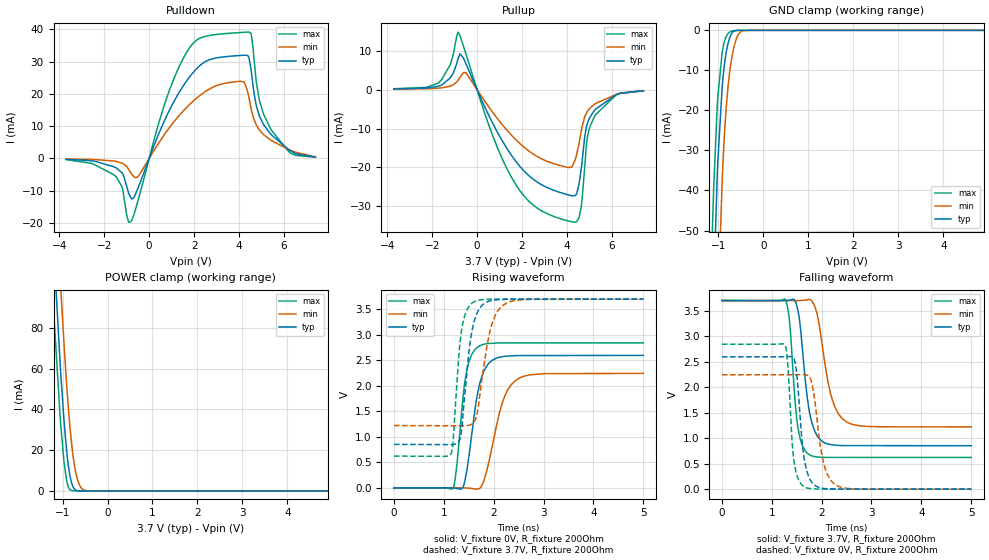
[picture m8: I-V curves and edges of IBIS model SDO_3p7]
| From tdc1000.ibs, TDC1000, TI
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|   Model
[Model]   SDO_3p7
Model_type   I/O
Polarity   Non-Inverting
Enable   Active-Low
Vinl = 1.11
Vinh = 2.59
Vmeas = 1.85
Vref = 0
Cref = 1pF
Rref = 100000
|   typ   min   max
C_comp   0.670pF   0.613pF   0.704pF
[Voltage Range]   3.7   3.699   3.701
[Temperature Range]   27   125   -40
[Pullup Reference]   3.7   3.699   3.701
[Pulldown Reference]   0   0   0
[Power Clamp Reference]   3.7   3.699   3.701
[GND Clamp Reference]   0   0   0
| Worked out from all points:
|   slope of the pulldown table from 0 to 0.555 V, typ, clamps not added: 57.1 ohm
|   slope of the pullup table from 0 to 0.555 V, typ, clamps not added: 79.3 ohm
|   GND clamp passes 1 mA (typ) near -0.71 V on its own axis
|   POWER clamp passes 1 mA (typ) near -0.74 V on its own axis
|   falling waveform, V_fixture 3.7V, R_fixture 200Ohm: 20-80 % time 197ps typ, 272ps min, 146ps max; typ from 3.7 V to 0.852 V
|   rising waveform, V_fixture 0V, R_fixture 200Ohm: 20-80 % time 241ps typ, 331ps min, 182ps max; typ from 0 V to 2.6 V
|   rising waveform, V_fixture 3.7V, R_fixture 200Ohm: 20-80 % time 193ps typ, 254ps min, 148ps max; typ from 0.852 V to 3.7 V
|   falling waveform, V_fixture 0V, R_fixture 200Ohm: 20-80 % time 148ps typ, 202ps min, 110ps max; typ from 2.6 V to 0 V
[Pulldown]
|   Voltage   I(typ)   I(min)   I(max)
-3.7V     -264.4uA   -158.9uA   -366.5uA
-1.491V   -2.825mA   -880.5uA   -5.512mA
-802.9mV  -12.37mA   -4.609mA   -19.5mA
640.1mV   11.08mA    7.012mA    15.79mA
1.728V    24.59mA    16.25mA    33.56mA
3.282V    31.44mA    23.14mA    38.61mA
4.381V    31.9mA     20.72mA    39.15mA
4.547V    26.85mA    15.15mA    38.38mA
4.769V    16.29mA    10.36mA    23.54mA
5.413V    7.511mA    5.656mA    9.091mA
6.334V    2.177mA    2.404mA    1.482mA
7.4V      424.2uA    504.5uA    390.1uA
[GND Clamp]
|   Voltage   I(typ)   I(min)   I(max)
-3.7V     -1.666A    -1.714A    -1.629A
-1.136V   -79.36mA   -127.2mA   -51.21mA
-1.125V   -74.22mA   -121.7mA   -46.88mA
-1.103V   -64.39mA   -110.8mA   -39mA
-1.014V   -33.13mA   -70.93mA   -16.92mA
-913.9mV  -13.9mA    -37.2mA    -5.349mA
-891.7mV  -11.24mA   -31.74mA   -4.004mA
-825.1mV  -5.503mA   -19.3mA    -1.54mA
-725.2mV  -1.216mA   -8.495mA   -302.2uA
-603.1mV  -61.85uA   -2.248mA   -21.83uA
-447.7mV  -847.8nA   -90.96uA   -178.6nA
7.4V      0A         0A         0A
[Pullup]
|   Voltage   I(typ)   I(min)   I(max)
-3.7V     166.1uA    103uA      227.5uA
-1.724V   857.1uA    384uA      1.69mA
-1.191V   3.033mA    905.6uA    6.459mA
-847.3mV  7.891mA    2.377mA    14.78mA
-492.1mV  6.622mA    4.285mA    9.107mA
640.1mV   -7.998mA   -5.394mA   -10.97mA
1.728V    -18.45mA   -12.87mA   -24.43mA
4.37V     -27.23mA   -17.96mA   -34.06mA
4.625V    -20.84mA   -11.02mA   -30.52mA
4.902V    -8.802mA   -5.659mA   -12.56mA
5.191V    -5.588mA   -3.907mA   -7.271mA
7.4V      -306.7uA   -312.1uA   -281.3uA
[POWER Clamp]
|   Voltage   I(typ)   I(min)   I(max)
-3.7V     1.442A     1.51A      1.381A
-1.236V   137.2mA    185.4mA    104.7mA
-1.202V   122.6mA    170.1mA    91mA
-1.18V    113.1mA    160mA      82.11mA
-1.036V   56.5mA     98.41mA    31.46mA
-969.4mV  35.13mA    73.03mA    14.76mA
-913.9mV  20.88mA    54.05mA    5.753mA
-814mV    5.313mA    26.64mA    318.7uA
-747.4mV  1.273mA    14.29mA    50.44uA
-669.7mV  118.2uA    5.73mA     8.141uA
-447.7mV  93.24nA    66.45uA    0A
7.4V      0A         0A         0A
[Ramp]
R_load = 200
|   typ   min   max
dV/dt_r   1.55786/2.40619e-10   1.34655/3.31006e-10   1.70581/1.8205e-10
dV/dt_f   1.70866/1.97079e-10   1.48608/2.72315e-10   1.84739/1.45755e-10
[Falling Waveform]
V_fixture = 3.7V
V_fixture_min = 3.699V
V_fixture_max = 3.701V
R_fixture = 200Ohm
C_fixture = 0F
|   Time   V(typ)   V(min)   V(max)
0s        3.7V       3.699V     3.701V
1.282ns   3.699V     3.698V     3.705V
1.366ns   3.709V     3.698V     3.201V
1.462ns   3.704V     3.698V     1.804V
1.519ns   3.53V      3.698V     1.247V
1.756ns   1.517V     3.722V     674mV
1.914ns   1.042V     3.418V     632.3mV
2.189ns   872.8mV    1.837V     623.4mV
2.418ns   855.7mV    1.379V     623.3mV
5ns       852.2mV    1.222V     622mV
[Rising Waveform]
V_fixture = 0V
V_fixture_min = 0V
V_fixture_max = 0V
R_fixture = 200Ohm
C_fixture = 0F
|   Time   V(typ)   V(min)   V(max)
0s        -769.6nV   -844.5nV   4.716uV
1.189ns   -4.254mV   637.4uV    1.645mV
1.253ns   -12.41mV   671.3uV    369.7mV
1.374ns   -6.095mV   318uV      1.66V
1.448ns   263.6mV    -2.92mV    2.233V
1.702ns   1.965V     -16.84mV   2.776V
1.908ns   2.447V     525.1mV    2.831V
2.174ns   2.572V     1.671V     2.841V
2.418ns   2.591V     2.09V      2.841V
5ns       2.596V     2.244V     2.843V
[Rising Waveform]
V_fixture = 3.7V
V_fixture_min = 3.699V
V_fixture_max = 3.701V
R_fixture = 200Ohm
C_fixture = 0F
|   Time   V(typ)   V(min)   V(max)
0s        852.2mV    1.222V     622mV
1.143ns   847.2mV    1.217V     664.7mV
1.186ns   848mV      1.217V     901.2mV
1.347ns   1.072V     1.217V     3.023V
1.505ns   2.671V     1.225V     3.561V
1.575ns   3.123V     1.256V     3.629V
1.681ns   3.457V     1.523V     3.672V
1.933ns   3.666V     3.102V     3.697V
2.174ns   3.692V     3.57V      3.7V
5ns       3.7V       3.699V     3.701V
[Falling Waveform]
|Gnd
V_fixture = 0V
V_fixture_min = 0V
V_fixture_max = 0V
R_fixture = 200Ohm
C_fixture = 0F
|   Time   V(typ)   V(min)   V(max)
0s        2.596V     2.244V     2.843V
1.266ns   2.599V     2.244V     2.832V
1.317ns   2.601V     2.244V     2.504V
1.448ns   2.557V     2.245V     538mV
1.505ns   2.225V     2.247V     274.9mV
1.651ns   602.7mV    2.247V     47.24mV
1.815ns   122.4mV    2.035V     6.36mV
2.055ns   11.69mV    455.7mV    852.2uV
2.268ns   2.035mV    92.15mV    790.5uV
5ns       -335.3nV   -872.9nV   -1.581uV
